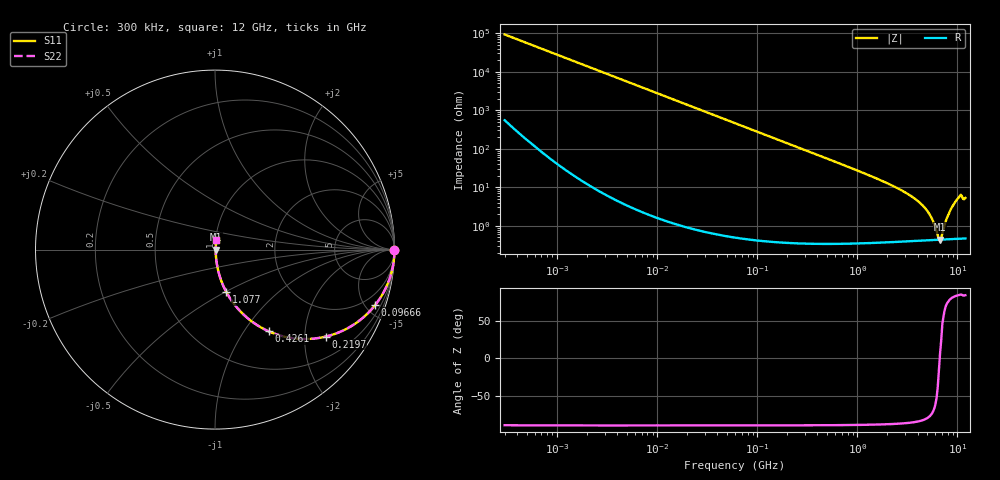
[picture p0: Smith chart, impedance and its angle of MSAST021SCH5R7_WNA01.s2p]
! MSAST021SCH5R7_WNA01  S-PARAMETER MODEL  ( General Type )
! Model Generated by TAIYO YUDEN Corporation (http://www.ty-top.com)
! Version 2.0
! TAIYO YUDEN Control No. 181101
! Copyright(c) 2015 TAIYO YUDEN CO.,LTD. All Rights Reserved.
! Product Description (link to TY-COMPAS)
! https://ds.yuden.co.jp/TYCOMPAS/or/detail?pn=MSAST021SCH5R7CWNA01&u=M
! Products Name : Multilayer Ceramic Capacitors
! Characteristics :
!  Capacitance : 5.7 pF , Rated Voltage : 25V , TCC : CH / C0H
!  Case Size : 0.25 x 0.125 / 0.0098 x 0.0049 [mm/inch] , Thickness : 0.125 / 0.0049 [mm/inch]
!  (Conditions: Temperature = 25 degC , DC Bias Current/Voltage = 0A / 0V)
! External Node Assignments :
!  1  o---| |---o  2
! GND o---------o GND
! Frequency Range : 0.3MHz  -  12000MHz  [ 401 STEP ]
# MHz S RI R 50
! Freq[MHz].  S11 Real  S11 Imag  S21 Real  S21 Imag  S12 Real  S12 Imag  S22 Real  S22 Imag
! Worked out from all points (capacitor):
!   401 points, 300 kHz to 12 GHz, reference 50 ohm
!   read as one part in series: C = 5.7 pF near 316.3 kHz
!   lowest |Z| = 440 mohm at 6.7 GHz (marker M1)
!   series resonance near 6.648 GHz, so ESL is about 100 pH
!   S11 on the Smith chart (normalised r, x): 300 kHz: open; 96.66 MHz: 1.01, -5.78; 219.7 MHz: 1.01, -2.54; 426.1 MHz: 1.01, -1.31; 1.077 GHz: 1.01, -0.50; 12 GHz: 1.01, +0.11
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0.3  1 -0.00107  7.53e-06 0.00107  7.53e-06 0.00107  1 -0.00107
1.769972  1 -0.00634  4.61e-05 0.00634  4.61e-05 0.00634  1 -0.00634
10.44266  0.9986 -0.0373  0.00142 0.0373  0.00142 0.0373  0.9986 -0.0373
27.82928  0.9901 -0.0987  0.00991 0.0987  0.00991 0.0987  0.9901 -0.0987
60  0.9557 -0.2053  0.0443 0.2053  0.0443 0.2053  0.9557 -0.2053
96.65937  0.8926 -0.3089  0.1074 0.3089  0.1074 0.3089  0.8926 -0.3089
219.7372  0.6167 -0.4848  0.3833 0.4848  0.3833 0.4848  0.6167 -0.4848
353.9943  0.3827 -0.4839  0.6173 0.4839  0.6173 0.4839  0.3827 -0.4839
426.1204  0.2996 -0.4555  0.7004 0.4555  0.7004 0.4555  0.2996 -0.4555
668.5285  0.148 -0.351  0.852 0.351  0.852 0.351  0.148 -0.351
1076.992  0.0628 -0.2357  0.9372 0.2357  0.9372 0.2357  0.0628 -0.2357
2088.533  0.0179 -0.1178  0.9821 0.1178  0.9821 0.1178  0.0179 -0.1178
3276.641  0.00803 -0.0636  0.992 0.0636  0.992 0.0636  0.00803 -0.0636
4502.883  0.00522 -0.033  0.9948 0.033  0.9948 0.033  0.00522 -0.033
5420.343  0.00452 -0.0168  0.9955 0.0168  0.9955 0.0168  0.00452 -0.0168
6354.153  0.00433 -0.00342  0.9957 0.00342  0.9957 0.00342  0.00433 -0.00342
6699.894  0.00435 0.000499  0.9956 -0.000499  0.9956 -0.000499  0.00435 0.000499
7064.448  0.0044 0.00459  0.9956 -0.00459  0.9956 -0.00459  0.0044 0.00459
8064.993  0.00478 0.0179  0.9952 -0.0179  0.9952 -0.0179  0.00478 0.0179
9207.246  0.00584 0.0361  0.9942 -0.0361  0.9942 -0.0361  0.00584 0.0361
10511.28  0.00791 0.0573  0.9921 -0.0573  0.9921 -0.0573  0.00791 0.0573
12000  0.00744 0.0523  0.9926 -0.0523  0.9926 -0.0523  0.00744 0.0523
